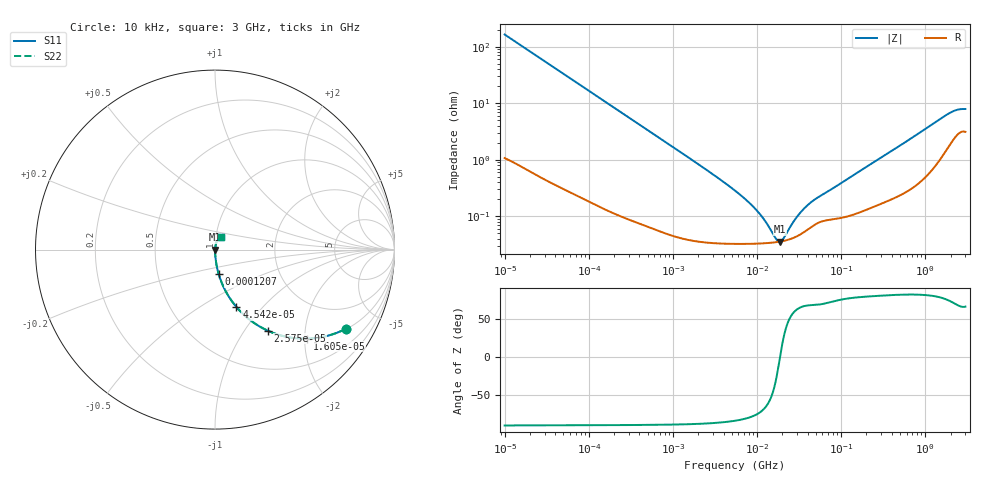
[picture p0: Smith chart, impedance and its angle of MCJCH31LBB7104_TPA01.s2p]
! MCJCH31LBB7104_TPA01  S-PARAMETER MODEL  ( Standard Model )
! Model Generated by TAIYO YUDEN Corporation (http://www.ty-top.com)
! Version 1.0
! TAIYO YUDEN Control No. 220601
! Copyright(c) 2015 TAIYO YUDEN CO.,LTD. All Rights Reserved.
! Product Description (link to TY-COMPAS)
! https://ds.yuden.co.jp/TYCOMPAS/or/detail?pn=MCJCH31LBB7104KTPA01&u=M
! Products Name : Multilayer Ceramic Capacitors
! Characteristics :
!  Capacitance : 0.1 [uF] , Rated Voltage : 100 [V] , TCC : X7R
!  Case Size : 3.2 x 1.6 / 0.126 x 0.063 [mm/inch] , Thickness : 1.6 / 0.063 [mm/inch]
!  (Conditions: Temperature = 25 [degC] , DC Bias Voltage = 0 [V])
! External Node Assignments :
!  1  o---| |---o  2
! GND o---------o GND
! Frequency Range : 10kHz  -  3GHz  [ 401 STEP ]
# MHZ S RI R 50
! Freq[MHz].  S11 Real  S11 Imag  S21 Real  S21 Imag  S12 Real  S12 Imag  S22 Real  S22 Imag
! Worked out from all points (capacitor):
!   401 points, 10 kHz to 3 GHz, reference 50 ohm
!   read as one part in series: C = 96.6 nF near 10.65 kHz
!   lowest |Z| = 35.9 mohm at 18.73 MHz (marker M1)
!   series resonance near 18.76 MHz, so ESL is about 750 pH
!   S11 on the Smith chart (normalised r, x): 10 kHz: 1.02, -3.29; 16.05 kHz: 1.01, -2.06; 25.75 kHz: 1.01, -1.28; 45.42 kHz: 1.01, -0.73; 120.7 kHz: 1.00, -0.28; 3 GHz: 1.06, +0.15
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0.01  0.729 -0.4412  0.271 0.4412  0.271 0.4412  0.729 -0.4412
0.016047  0.5137 -0.4962  0.4863 0.4962  0.4863 0.4962  0.5137 -0.4962
0.02575  0.2934 -0.4514  0.7066 0.4514  0.7066 0.4514  0.2934 -0.4514
0.045421  0.1197 -0.3202  0.8803 0.3202  0.8803 0.3202  0.1197 -0.3202
0.082683  0.0408 -0.1926  0.9592 0.1926  0.9592 0.1926  0.0408 -0.1926
0.120707  0.0202 -0.1351  0.9798 0.1351  0.9798 0.1351  0.0202 -0.1351
0.257252  0.00517 -0.0647  0.9948 0.0647  0.9948 0.0647  0.00517 -0.0647
0.683653  0.00116 -0.0246  0.9988 0.0246  0.9988 0.0246  0.00116 -0.0246
5.477226  0.000334 -0.00284  0.9997 0.00284  0.9997 0.00284  0.000334 -0.00284
9.97066  0.000331 -0.00122  0.9997 0.00122  0.9997 0.00122  0.000331 -0.00122
12.43293  0.000336 -0.000768  0.9997 0.000768  0.9997 0.000768  0.000336 -0.000768
16.51234  0.000349 -0.000232  0.9997 0.000232  0.9997 0.000232  0.000349 -0.000232
17.5871  0.000353 -0.000117  0.9996 0.000117  0.9996 0.000117  0.000353 -0.000117
18.73182  0.000358 -2.24e-06  0.9996 2.24e-06  0.9996 2.24e-06  0.000358 -2.24e-06
20.5901  0.000368 0.00017  0.9996 -0.00017  0.9996 -0.00017  0.000368 0.00017
26.49725  0.000411 0.000642  0.9996 -0.000642  0.9996 -0.000642  0.000411 0.000642
32.0153  0.000471 0.00102  0.9995 -0.00102  0.9995 -0.00102  0.000471 0.00102
45.28751  0.000669 0.00172  0.9993 -0.00172  0.9993 -0.00172  0.000669 0.00172
374.4521  0.0021 0.0133  0.9979 -0.0133  0.9979 -0.0133  0.0021 0.0133
1869.516  0.02 0.0605  0.98 -0.0605  0.98 -0.0605  0.02 0.0605
2331.196  0.0303 0.0672  0.9697 -0.0672  0.9697 -0.0672  0.0303 0.0672
3000  0.0351 0.0681  0.9649 -0.0681  0.9649 -0.0681  0.0351 0.0681
